| TEXAS INSTRUMENTS INCORPORATED
| Standard Linear and Logic Group
| IBIS Model of SN74CB3Q16210
| 20 Bit Switch 2.5V/3.3V Low-Voltage FET Bus Switch
| This file contains package information for the following:
|  TSSOP 48-pin (DGG) package as [Component] CB3Q16210_DGG
|  TVSOP 48-pin (DGV) package as [Component] CB3Q16210_DGV
|  SSOP 48-pin (DL) package as [Component] CB3Q16210_DL
| This device can be powered at the following Vccs:
|  3.3 volt Vcc
|  2.5 volt Vcc
| This file provides unique models under the [Model Selector] for each Vcc.
| For operation at a specific Vcc, select the appropriate model after each
| [Model Selector] keyword.
[IBIS Ver]   3.2
[Comment char]  |_char
[File Name]   sn74cb3q16210.ibs
[File Rev]   1.1 | a_die
[Date]   April 30, 2004
[Source]   Data created from TI-SPICE simulations at TI-SLL.
[Notes]   The following is an IBIS list for the CB3Q16210.
   Please contact sllibis@ti.com with questions and
   comments concerning SLL IBIS models.
   - FILE REV HISTORY
   - 1.1 Release IBIS file on 05/05/04
   - Power clamp data deleted as there is no power-clamp diode
[Disclaimer] Property of Texas Instruments Incorporated.  Unauthorized
   reproduction and/or distribution is strictly prohibited.
   This product is protected under copyright law.
   Created  2003, (C) Copyright  2003, Texas Instruments
   Incorporated, All Rights Reserved
   UNLESS THERE IS A SIGNED, WRITTEN AGREEMENT TO THE
   CONTRARY, TEXAS INSTRUMENTS (TI) IS PROVIDING THE IBIS
   MODELS  AND WITHOUT ANY WARRANTY, EXPRESSED OR
   IMPLIED.  TI assumes no liability for:
   1) the accuracy of the IBIS models provided to your
   company;
   2) the proper functioning of these IBIS Models in your
   design or for any resulting applications; or
   3) infringement of patents, copyrights or intellectual
   property rights resulting from your use of these IBIS
   models.
   TI provides IBIS Models as a service to our customers.
   You and your company shall not distribute, sell or give
   these models to anyone else without prior written
   permission from TI.
   TI reserves the right to make changes to our products or
   to discontinue any semiconductor product or service
   without notice, and advises our customers to obtain the
   latest version of relevant information to verify, before
   placing orders, that the information being relied on is
   current.
   Please be aware that your receipt and use of the IBIS
   information provided shall serve as acceptance of these
   terms and conditions.  If you do not accept these terms,
   you should return or destroy the IBIS models and any
   other accompanying information immediately.
| Component CB3Q16210_DGG 48-pin TSSOP
[Component]   CB3Q16210_DGG
[Manufacturer]   Texas Instruments, Inc.
[Package]
|   typ   min   max
R_pkg   6.200e-02   5.000e-02   7.800e-02
L_pkg   3.527e-09   3.128e-09   4.255e-09
C_pkg   5.300e-13   4.170e-13   6.850e-13
[Pin]   signal_name   model_name   R_pin   L_pin   C_pin
1   NC   NC   5.000e-02   4.250e-09   6.710e-13
2   1A1   CB3Q16210_IO   5.700e-02   3.956e-09   6.740e-13
3   1A2   CB3Q16210_IO   7.100e-02   3.922e-09   6.190e-13
4   1A3   CB3Q16210_IO   7.800e-02   3.841e-09   6.180e-13
5   1A4   CB3Q16210_IO   5.600e-02   3.535e-09   5.550e-13
6   1A5   CB3Q16210_IO   5.800e-02   3.464e-09   5.030e-13
7   1A6   CB3Q16210_IO   6.000e-02   3.362e-09   4.980e-13
8   GND   GND   6.100e-02   3.293e-09   4.620e-13
9   1A7   CB3Q16210_IO   6.300e-02   3.240e-09   4.550e-13
10   1A8   CB3Q16210_IO   6.300e-02   3.175e-09   4.420e-13
11   1A9   CB3Q16210_IO   6.400e-02   3.153e-09   4.290e-13
12   1A10   CB3Q16210_IO   6.500e-02   3.128e-09   4.180e-13
13   2A1   CB3Q16210_IO   6.500e-02   3.128e-09   4.180e-13
14   2A2   CB3Q16210_IO   6.400e-02   3.154e-09   4.290e-13
15   VCC   POWER   6.300e-02   3.174e-09   4.420e-13
16   2A3   CB3Q16210_IO   6.300e-02   3.241e-09   4.550e-13
17   GND   GND   6.100e-02   3.293e-09   4.620e-13
18   2A4   CB3Q16210_IO   6.000e-02   3.362e-09   4.970e-13
19   2A5   CB3Q16210_IO   5.800e-02   3.464e-09   5.030e-13
20   2A6   CB3Q16210_IO   5.600e-02   3.537e-09   5.600e-13
21   2A7   CB3Q16210_IO   7.700e-02   3.839e-09   6.260e-13
22   2A8   CB3Q16210_IO   7.100e-02   3.917e-09   6.270e-13
23   2A9   CB3Q16210_IO   5.800e-02   3.955e-09   6.850e-13
24   2A10   CB3Q16210_IO   5.200e-02   4.255e-09   6.790e-13
25   2B10   CB3Q16210_IO   5.100e-02   4.254e-09   6.760e-13
26   2B9   CB3Q16210_IO   5.800e-02   3.957e-09   6.790e-13
27   2B8   CB3Q16210_IO   7.100e-02   3.920e-09   6.210e-13
28   2B7   CB3Q16210_IO   7.800e-02   3.843e-09   6.220e-13
29   2B6   CB3Q16210_IO   5.600e-02   3.539e-09   5.600e-13
30   2B5   CB3Q16210_IO   5.800e-02   3.466e-09   5.030e-13
31   2B4   CB3Q16210_IO   6.000e-02   3.363e-09   4.970e-13
32   GND   GND   6.100e-02   3.294e-09   4.620e-13
33   2B3   CB3Q16210_IO   6.300e-02   3.241e-09   4.540e-13
34   2B2   CB3Q16210_IO   6.300e-02   3.175e-09   4.410e-13
35   2B1   CB3Q16210_IO   6.400e-02   3.153e-09   4.290e-13
36   1B10   CB3Q16210_IO   6.500e-02   3.129e-09   4.170e-13
37   1B9   CB3Q16210_IO   6.500e-02   3.129e-09   4.170e-13
38   1B8   CB3Q16210_IO   6.400e-02   3.152e-09   4.290e-13
39   1B7   CB3Q16210_IO   6.400e-02   3.176e-09   4.410e-13
40   1B6   CB3Q16210_IO   6.300e-02   3.241e-09   4.540e-13
41   GND   GND   6.100e-02   3.293e-09   4.620e-13
42   1B5   CB3Q16210_IO   6.000e-02   3.363e-09   4.970e-13
43   1B4   CB3Q16210_IO   5.800e-02   3.464e-09   5.030e-13
44   1B3   CB3Q16210_IO   5.600e-02   3.534e-09   5.610e-13
45   1B2   CB3Q16210_IO   7.800e-02   3.841e-09   6.260e-13
46   1B1   CB3Q16210_IO   7.100e-02   3.920e-09   6.220e-13
47   2NOE   CB3Q16210_IN   5.700e-02   3.955e-09   6.770e-13
48   1NOE   CB3Q16210_IN   5.100e-02   4.252e-09   6.720e-13
| Component CB3Q16210_DGV 48-pin TVSOP
[Component]   CB3Q16210_DGV
[Manufacturer]   Texas Instruments, Inc.
[Package]
|   typ   min   max
R_pkg   7.000e-02   4.900e-02   8.500e-02
L_pkg   3.013e-09   2.743e-09   3.408e-09
C_pkg   3.710e-13   2.940e-13   5.110e-13
[Pin]   signal_name   model_name   R_pin   L_pin   C_pin
1   NC   NC   4.900e-02   3.393e-09   4.970e-13
2   1A1   CB3Q16210_IO   6.000e-02   3.250e-09   5.020e-13
3   1A2   CB3Q16210_IO   7.700e-02   3.310e-09   4.510e-13
4   1A3   GND   8.500e-02   3.299e-09   4.040e-13
5   1A4   CB3Q16210_IO   8.300e-02   3.136e-09   3.600e-13
6   1A5   CB3Q16210_IO   7.700e-02   3.019e-09   3.630e-13
7   1A6   POWER   6.500e-02   2.882e-09   3.490e-13
8   GND   CB3Q16210_IO   6.600e-02   2.829e-09   3.140e-13
9   1A7   CB3Q16210_IO   6.700e-02   2.796e-09   3.140e-13
10   1A8   GND   6.900e-02   2.754e-09   3.080e-13
11   1A9   CB3Q16210_IO   7.000e-02   2.753e-09   3.010e-13
12   1A10   CB3Q16210_IO   7.100e-02   2.745e-09   2.940e-13
13   2A1   CB3Q16210_IO   7.000e-02   2.744e-09   2.940e-13
14   2A2   CB3Q16210_IO   7.000e-02   2.754e-09   3.010e-13
15   VCC   GND   6.900e-02   2.754e-09   3.080e-13
16   2A3   CB3Q16210_IO   6.700e-02   2.796e-09   3.140e-13
17   GND   CB3Q16210_IO   6.600e-02   2.829e-09   3.140e-13
18   2A4   POWER   6.500e-02   2.883e-09   3.500e-13
19   2A5   CB3Q16210_IO   7.500e-02   3.014e-09   3.630e-13
20   2A6   CB3Q16210_IO   8.000e-02   3.128e-09   3.580e-13
21   2A7   GND   8.400e-02   3.295e-09   4.030e-13
22   2A8   CB3Q16210_IO   7.800e-02   3.311e-09   4.520e-13
23   2A9   CB3Q16210_IO   6.200e-02   3.259e-09   5.010e-13
24   2A10   CB3Q16210_IO   5.200e-02   3.404e-09   4.960e-13
25   2B10   CB3Q16210_IO   5.300e-02   3.397e-09   5.050e-13
26   2B9   CB3Q16210_IO   6.200e-02   3.249e-09   5.110e-13
27   2B8   CB3Q16210_IO   7.700e-02   3.308e-09   4.530e-13
28   2B7   GND   8.200e-02   3.289e-09   4.030e-13
29   2B6   CB3Q16210_IO   7.800e-02   3.121e-09   3.590e-13
30   2B5   CB3Q16210_IO   7.400e-02   3.010e-09   3.630e-13
31   2B4   POWER   6.500e-02   2.883e-09   3.490e-13
32   GND   CB3Q16210_IO   6.700e-02   2.829e-09   3.140e-13
33   2B3   CB3Q16210_IO   6.700e-02   2.795e-09   3.140e-13
34   2B2   GND   6.900e-02   2.753e-09   3.070e-13
35   2B1   CB3Q16210_IO   7.000e-02   2.753e-09   3.010e-13
36   1B10   CB3Q16210_IO   7.000e-02   2.743e-09   2.940e-13
37   1B9   CB3Q16210_IO   7.000e-02   2.743e-09   2.940e-13
38   1B8   CB3Q16210_IO   7.000e-02   2.753e-09   3.010e-13
39   1B7   GND   6.900e-02   2.754e-09   3.070e-13
40   1B6   CB3Q16210_IO   6.800e-02   2.797e-09   3.140e-13
41   GND   CB3Q16210_IO   6.700e-02   2.830e-09   3.140e-13
42   1B5   POWER   6.400e-02   2.880e-09   3.490e-13
43   1B4   CB3Q16210_IO   7.200e-02   3.004e-09   3.620e-13
44   1B3   CB3Q16210_IO   7.800e-02   3.121e-09   3.590e-13
45   1B2   GND   8.400e-02   3.296e-09   4.030e-13
46   1B1   CB3Q16210_IO   7.700e-02   3.308e-09   4.510e-13
47   2NOE   CB3Q16210_IN   6.200e-02   3.258e-09   4.990e-13
48   1NOE   CB3Q16210_IN   5.300e-02   3.408e-09   4.940e-13
| Component CB3Q16210_DL 48-pin SSOP
[Component]   CB3Q16210_DL
[Manufacturer]   Texas Instruments, Inc.
[Package]
|   typ   min   max
R_pkg   4.800e-02   3.800e-02   5.300e-02
L_pkg   6.046e-09   5.084e-09   7.968e-09
C_pkg   8.130e-13   5.690e-13   1.157e-12
[Pin]   signal_name   model_name   R_pin   L_pin   C_pin
1   NC   NC   4.600e-02   7.968e-09   1.017e-12
2   1A1   CB3Q16210_IO   4.400e-02   7.299e-09   1.157e-12
3   1A2   CB3Q16210_IO   4.300e-02   6.765e-09   1.058e-12
4   1A3   GND   4.100e-02   6.269e-09   9.330e-13
5   1A4   CB3Q16210_IO   3.800e-02   5.856e-09   8.290e-13
6   1A5   CB3Q16210_IO   4.600e-02   5.802e-09   7.900e-13
7   1A6   POWER   5.000e-02   5.656e-09   7.380e-13
8   GND   CB3Q16210_IO   5.300e-02   5.500e-09   6.430e-13
9   1A7   CB3Q16210_IO   5.200e-02   5.304e-09   6.060e-13
10   1A8   GND   5.300e-02   5.189e-09   5.830e-13
11   1A9   CB3Q16210_IO   5.100e-02   5.084e-09   5.690e-13
12   1A10   CB3Q16210_IO   5.300e-02   5.862e-09   8.330e-13
13   2A1   CB3Q16210_IO   5.300e-02   5.862e-09   8.330e-13
14   2A2   CB3Q16210_IO   5.100e-02   5.084e-09   5.690e-13
15   VCC   GND   5.300e-02   5.189e-09   5.830e-13
16   2A3   CB3Q16210_IO   5.200e-02   5.304e-09   6.060e-13
17   GND   CB3Q16210_IO   5.300e-02   5.500e-09   6.430e-13
18   2A4   POWER   5.000e-02   5.656e-09   7.380e-13
19   2A5   CB3Q16210_IO   4.600e-02   5.802e-09   7.900e-13
20   2A6   CB3Q16210_IO   3.800e-02   5.856e-09   8.290e-13
21   2A7   GND   4.100e-02   6.269e-09   9.330e-13
22   2A8   CB3Q16210_IO   4.300e-02   6.765e-09   1.058e-12
23   2A9   CB3Q16210_IO   4.400e-02   7.299e-09   1.157e-12
24   2A10   CB3Q16210_IO   4.600e-02   7.968e-09   1.017e-12
25   2B10   CB3Q16210_IO   4.600e-02   7.968e-09   1.017e-12
26   2B9   CB3Q16210_IO   4.400e-02   7.299e-09   1.157e-12
27   2B8   CB3Q16210_IO   4.300e-02   6.765e-09   1.058e-12
28   2B7   GND   4.100e-02   6.269e-09   9.330e-13
29   2B6   CB3Q16210_IO   3.800e-02   5.856e-09   8.290e-13
30   2B5   CB3Q16210_IO   4.600e-02   5.802e-09   7.900e-13
31   2B4   POWER   5.000e-02   5.656e-09   7.380e-13
32   GND   CB3Q16210_IO   5.300e-02   5.500e-09   6.430e-13
33   2B3   CB3Q16210_IO   5.200e-02   5.304e-09   6.060e-13
34   2B2   GND   5.300e-02   5.189e-09   5.830e-13
35   2B1   CB3Q16210_IO   5.100e-02   5.084e-09   5.690e-13
36   1B10   CB3Q16210_IO   5.300e-02   5.862e-09   8.330e-13
37   1B9   CB3Q16210_IO   5.300e-02   5.862e-09   8.330e-13
38   1B8   CB3Q16210_IO   5.100e-02   5.084e-09   5.690e-13
39   1B7   GND   5.300e-02   5.189e-09   5.830e-13
40   1B6   CB3Q16210_IO   5.200e-02   5.304e-09   6.060e-13
41   GND   CB3Q16210_IO   5.300e-02   5.500e-09   6.430e-13
42   1B5   POWER   5.000e-02   5.656e-09   7.380e-13
43   1B4   CB3Q16210_IO   4.600e-02   5.802e-09   7.900e-13
44   1B3   CB3Q16210_IO   3.800e-02   5.856e-09   8.290e-13
45   1B2   GND   4.100e-02   6.269e-09   9.330e-13
46   1B1   CB3Q16210_IO   4.300e-02   6.765e-09   1.058e-12
47   2NOE   CB3Q16210_IN   4.400e-02   7.299e-09   1.157e-12
48   1NOE   CB3Q16210_IN   4.600e-02   7.967e-09   1.017e-12
[Series Switch Groups]
| Function Group States
On  1 /   | 1A1-1A10->1B1-1B10 1NOE LOW
On  2 /   | 2A1-2A10->2B1-2B10 2NOE LOW
On  1 2  /   | Enable Both
[Series Pin Mapping]   pin_2   model_name   function_table_group
2   46   CB3Q16210_IO_33_S   1
| 2   46   CB3Q16210_IO_25_S   1
3   45   CB3Q16210_IO_33_S   1
| 3   45   CB3Q16210_IO_25_S   1
4   44   CB3Q16210_IO_33_S   1
| 4   44   CB3Q16210_IO_25_S   1
5   43   CB3Q16210_IO_33_S   1
| 5   43   CB3Q16210_IO_25_S   1
6   42   CB3Q16210_IO_33_S   1
| 6   42   CB3Q16210_IO_25_S   1
7   40   CB3Q16210_IO_33_S   1
| 7   40   CB3Q16210_IO_25_S   1
9   39   CB3Q16210_IO_33_S   1
| 9   39   CB3Q16210_IO_25_S   1
10   38   CB3Q16210_IO_33_S   1
| 10   38   CB3Q16210_IO_25_S   1
11   37   CB3Q16210_IO_33_S   1
| 11   37   CB3Q16210_IO_25_S   1
12   36   CB3Q16210_IO_33_S   1
| 12   36   CB3Q16210_IO_25_S   1
13   35   CB3Q16210_IO_33_S   2
| 13   35   CB3Q16210_IO_25_S   2
14   34   CB3Q16210_IO_33_S   2
| 14   34   CB3Q16210_IO_25_S   2
16   33   CB3Q16210_IO_33_S   2
| 16   33   CB3Q16210_IO_25_S   2
18   31   CB3Q16210_IO_33_S   2
| 18   31   CB3Q16210_IO_25_S   2
19   30   CB3Q16210_IO_33_S   2
| 19   30   CB3Q16210_IO_25_S   2
20   29   CB3Q16210_IO_33_S   2
| 20   29   CB3Q16210_IO_25_S   2
21   28   CB3Q16210_IO_33_S   2
| 21   28   CB3Q16210_IO_25_S   2
22   27   CB3Q16210_IO_33_S   2
| 22   27   CB3Q16210_IO_25_S   2
23   26   CB3Q16210_IO_33_S   2
| 23   26   CB3Q16210_IO_25_S   2
24   25   CB3Q16210_IO_33_S   2
| 24   25   CB3Q16210_IO_25_S   2
| Model CB3Q16210_IN
[Model Selector]   CB3Q16210_IN
CB3Q16210_IN_33   3.3 volt Vcc
CB3Q16210_IN_25   2.5 volt Vcc
| Model CB3Q16210_IO
[Model Selector]   CB3Q16210_IO
CB3Q16210_IO_33   3.3 volt Vcc
CB3Q16210_IO_25   2.5 volt Vcc
| Model CB3Q16210_IO_S
[Model Selector]   CB3Q16210_IO_S
CB3Q16210_IO_33_S   3.3 volt Vcc_S
CB3Q16210_IO_25_S   2.5 volt Vcc_S
[Model]   CB3Q16210_IO_33_S
Model_type  Series_switch
| variable   typ   min   max
C_comp   0   0   0
[Temperature Range]   40   100   -40
| Ambient temperature   25   85   -40
[Voltage range]   3.3   3   3.6
[On]
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[Off]
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[Model]   CB3Q16210_IO_25_S
Model_type  Series_switch
| variable   typ   min   max
C_comp   0   0   0
[Temperature Range]   40   100   -40
| Ambient temperature   25   85   -40
[Voltage range]   2.5   2.3   2.7
[On]
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[Off]
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| Models and submodels in the file (6): CB3Q16210_IN_33 (Input), CB3Q16210_IN_25 (Input), CB3Q16210_IO_33_S (Series_switch), CB3Q16210_IO_33 (Terminator), CB3Q16210_IO_25_S (Series_switch), CB3Q16210_IO_25 (Terminator)
